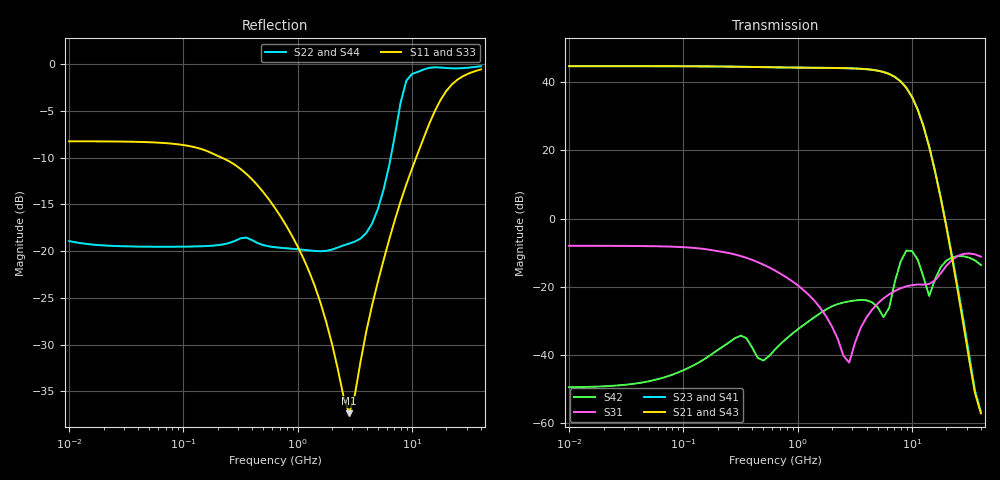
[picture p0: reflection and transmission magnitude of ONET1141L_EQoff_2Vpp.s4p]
! Touchstone Ver. 1.0
! Fri Mar 23 19:24:49 2012
! Number of ports is 4
# Hz	S	DB	R	50.000000
! SCATTERING PARAMETERS  :
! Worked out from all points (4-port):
!   73 points, 10 MHz to 40 GHz, reference 50 ohm
!   strongest paths, dB at 10 MHz, 79.43 MHz, 631 MHz, 5.012 GHz, 40 GHz:
!     S21: 44.6, 44.6, 44.3, 43.3, -57.1
!     S23: 44.6, 44.6, 44.3, 43.3, -56.6
!     S41: 44.6, 44.6, 44.3, 43.3, -56.7
!     S43: 44.6, 44.6, 44.3, 43.3, -56.9
!     S31: -8.0, -8.2, -15.2, -24.9, -11.2
!     S42: -49.4, -45.8, -38.4, -26.0, -13.6
!   lowest |S11| = -37.3 dB at 2.818 GHz (marker M1), VSWR 1.03, Z = 48.7 - j0.172 ohm
!   |S11| at or under -10 dB: 215.9 MHz to 10.88 GHz (10.66 GHz wide, 192 % of centre)
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1e7  -8.25 -2.0  -109.25 92.2  -8.00 -1.7  -108.73 92.7
     44.62 -177.8  -18.92 24.6  44.62 2.2  -49.17 12.8
     -8.00 -1.7  -109.03 92.0  -8.26 -2.0  -108.90 93.7
     44.61 2.2  -49.42 12.9  44.61 -177.8  -18.93 24.6
7.079458e8  -16.29 -73.0  -54.43 96.9  -16.11 -68.7  -54.46 96.9
            44.26 151.2  -19.64 -15.7  44.26 -28.8  -36.90 70.0
            -16.18 -68.5  -54.42 96.8  -16.22 -73.2  -54.43 96.8
            44.26 -28.8  -36.74 68.0  44.26 151.2  -19.60 -15.6
2.818383e9  -37.34 -172.5  -43.86 -6.3  -42.60 32.2  -43.86 -6.3
            44.00 69.1  -19.19 -61.9  44.00 -110.9  -23.56 36.8
            -42.21 18.1  -43.85 -6.4  -36.65 -177.7  -43.85 -6.3
            44.00 -111.0  -24.26 37.4  43.99 69.0  -19.17 -64.7
4.466836e9  -25.81 104.9  -45.82 -34.9  -26.19 64.7  -45.80 -35.1
            43.56 1.6  -17.06 -121.0  43.57 -178.4  -24.03 3.1
            -26.71 64.1  -45.81 -35.0  -25.46 103.8  -45.81 -34.8
            43.56 -178.7  -24.52 5.1  43.55 1.4  -17.02 -122.8
6.309573e9  -18.77 85.9  -45.20 -52.7  -22.06 52.5  -45.17 -53.0
            42.34 -78.0  -10.84 -178.6  42.36 102.1  -26.39 -121.0
            -22.19 55.9  -45.18 -52.3  -18.92 83.9  -45.18 -52.0
            42.35 101.7  -26.17 -140.1  42.32 -78.3  -10.43 179.4
1e10  -11.17 50.1  -44.16 -133.9  -19.44 44.3  -44.05 -134.4
      35.55 117.6  -1.05 67.7  35.63 -62.3  -8.98 46.2
      -19.51 42.9  -43.94 -134.2  -11.18 50.8  -43.98 -134.0
      35.55 -62.7  -9.51 45.0  35.46 117.4  -1.25 67.6
4e10  -0.57 -107.5  -58.86 2.2  -11.16 -16.4  -58.59 1.2
      -57.06 -13.5  -0.22 -118.6  -56.63 48.8  -13.60 -28.1
      -11.16 -16.4  -58.69 1.6  -0.57 -107.4  -58.71 1.9
      -56.65 47.9  -13.60 -28.1  -56.93 -13.1  -0.22 -118.6
